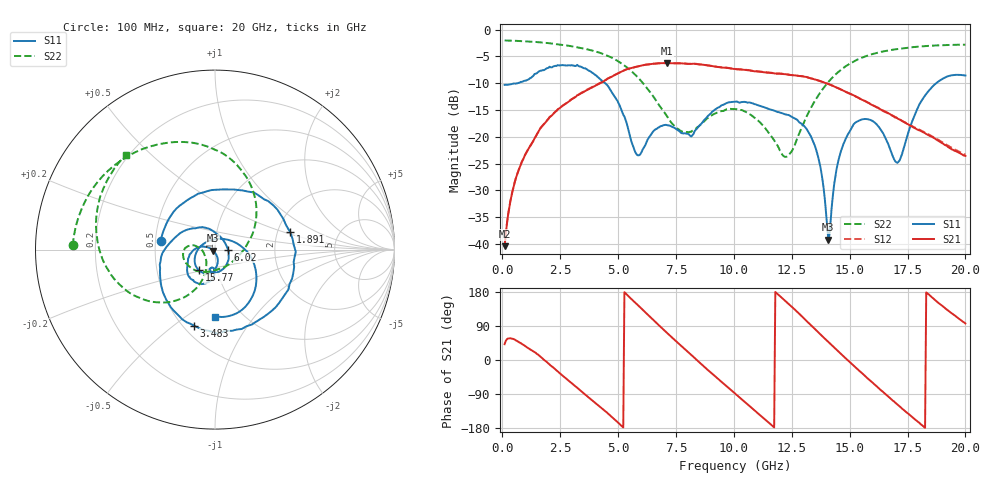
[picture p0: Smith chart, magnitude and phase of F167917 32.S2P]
!  2-Port S-parameters saved by WinCal
! VAR MeasName=S-Parameters (CALIBRATED_DATA) read from VNA (N5242A)
! VAR MeasDate=2016-11-22 9:01:17
! VAR NAME=F167917 32
! VAR FILENAME=F167917 32.S2P
! VAR DATE=2016-11-22 9:01:17
! VAR PHYS_PORTS=1,2
# Hz S DB R 50
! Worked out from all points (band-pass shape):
!   401 points, 100 MHz to 20 GHz, reference 50 ohm
!   highest |S21| = -6.24 dB at 7.115 GHz (marker M1); lowest = -40.4 dB at 100 MHz (marker M2)
!   |S21| within 3 dB of the highest: 4.525 GHz to 13.44 GHz (8.919 GHz wide, 99.3 % of centre)
!   lowest |S11| = -39.2 dB at 14.08 GHz (marker M3), VSWR 1.02, Z = 49.1 - j0.594 ohm
!   |S11| at or under -10 dB: start of sweep to 662.5 MHz; 4.444 GHz to 18.74 GHz (14.29 GHz wide, 123 % of centre)
!   |S22| runs from -23.8 to -2.0 dB; largest |S21 - S12| = 0.0035
!   S11 on the Smith chart (normalised r, x): 100 MHz: 0.54, +0.06; 1.891 GHz: 2.36, +0.56; 3.483 GHz: 0.57, -0.60; 6.02 GHz: 1.16, +0.00; 15.77 GHz: 0.81, -0.19; 20 GHz: 0.76, -0.66
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1e8  -10.32 170.8  -40.43 41.8  -40.37 42.0  -2.03 178.3
6.97e8  -9.96 115.6  -26.33 47.9  -26.31 47.7  -2.12 168.4
1.891e9  -7.30 12.9  -17.21 -3.7  -17.22 -3.7  -2.48 148.5
2.687e9  -6.67 -50.9  -13.97 -45.6  -13.95 -45.4  -2.90 134.3
3.43325e9  -7.03 -102.1  -11.84 -83.7  -11.77 -83.7  -3.47 119.7
3.483e9  -7.13 -105.2  -11.72 -86.2  -11.64 -86.2  -3.52 118.6
5.02525e9  -13.75 150.6  -8.10 -166.6  -8.09 -167.0  -5.96 78.6
6.02025e9  -22.79 0.4  -6.69 135.1  -6.70 135.0  -9.72 45.0
6.7665e9  -18.25 -76.3  -6.28 91.5  -6.28 91.5  -14.09 14.9
7.11475e9  -17.84 -93.3  -6.24 71.5  -6.25 71.6  -16.19 -3.1
8.458e9  -18.21 -91.1  -6.47 -3.3  -6.45 -3.2  -18.13 -102.7
1.005e10  -13.47 -121.0  -7.35 -88.2  -7.33 -88.1  -14.85 -168.3
1.1244e10  -14.40 -144.8  -7.94 -151.3  -7.89 -151.2  -17.83 169.0
1.2239e10  -15.82 -158.4  -8.33 154.9  -8.31 154.7  -23.77 -158.0
1.338325e10  -20.47 172.3  -9.14 88.6  -9.16 88.8  -14.18 -113.2
1.407975e10  -39.21 -146.5  -10.13 47.7  -10.16 47.8  -9.80 -123.7
1.47265e10  -21.44 -81.5  -11.37 10.2  -11.36 10.5  -7.17 -137.9
1.577125e10  -16.72 -128.1  -13.61 -48.3  -13.58 -47.6  -4.86 -161.0
1.67165e10  -21.94 164.6  -15.70 -99.0  -15.73 -98.5  -3.86 -179.0
1.716425e10  -24.38 80.4  -16.79 -122.8  -16.78 -122.2  -3.58 173.5
1.8408e10  -11.48 -30.6  -19.73 173.6  -19.56 173.9  -3.04 154.7
2e10  -8.57 -89.6  -23.58 96.5  -23.36 96.5  -2.82 133.2
